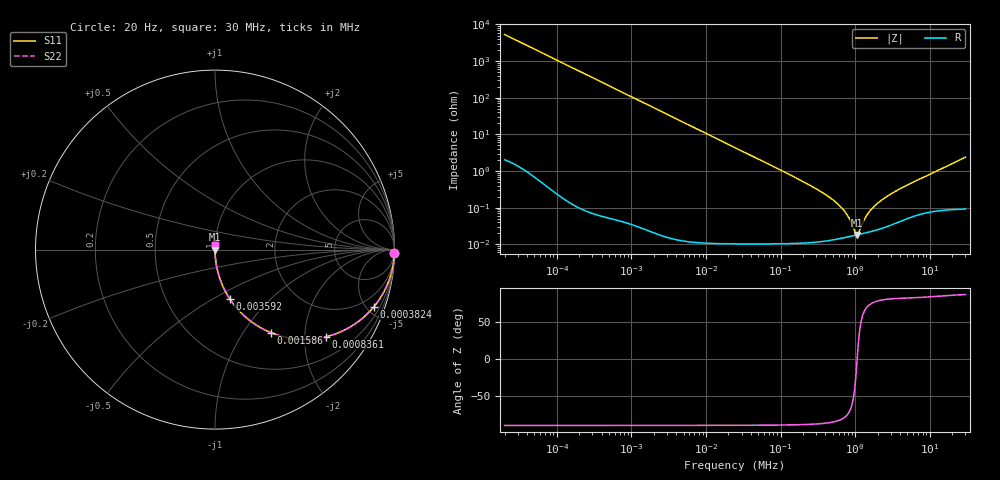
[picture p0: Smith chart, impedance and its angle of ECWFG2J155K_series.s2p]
!  *** S-Parameter ***
!  Copyright (C) Panasonic Industry
!  Plastic Film Capacitor (ECWFG)
!  Parts No. ECWFG2J155K
!  Connection Mode : Series
!  1  o---||---o  2
!  GND o--------o GND
!  Conditions : Temperature = 20   DC Bias = 0 V
! Frequency Range : 20 Hz  -  30 MHz  [ 401 Steps ]
# Hz S RI R 50
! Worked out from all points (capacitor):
!   401 points, 20 Hz to 30 MHz, reference 50 ohm
!   read as one part in series: C = 1.49 uF near 21.47 Hz
!   lowest |Z| = 18.1 mohm at 1.061 MHz (marker M1)
!   series resonance near 1.062 MHz, so ESL is about 15 nH
!   S11 on the Smith chart (normalised r, x): 20 Hz: open; 382.4 Hz: 1.00, -5.58; 836.1 Hz: 1.00, -2.55; 1.586 kHz: 1.00, -1.35; 3.592 kHz: 1.00, -0.59; 30 MHz: 1.00, +0.05
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20  0.9996 -0.0187  0.000358 0.0187  0.000358 0.0187  0.9996 -0.0187
80.02006  0.9944 -0.0745  0.00561 0.0745  0.00561 0.0745  0.9944 -0.0745
216.5336  0.9604 -0.1948  0.0396 0.1948  0.0396 0.1948  0.9604 -0.1948
382.445  0.8862 -0.3175  0.1138 0.3175  0.1138 0.3175  0.8862 -0.3175
836.0918  0.6198 -0.4853  0.3802 0.4853  0.3802 0.4853  0.6198 -0.4853
1585.543  0.3121 -0.4632  0.6879 0.4632  0.6879 0.4632  0.3121 -0.4632
2344.34  0.1719 -0.3771  0.8281 0.3771  0.8281 0.3771  0.1719 -0.3771
3591.727  0.0813 -0.2731  0.9187 0.2731  0.9187 0.2731  0.0813 -0.2731
8430.8  0.0159 -0.1246  0.9841 0.1246  0.9841 0.1246  0.0159 -0.1246
24494.9  0.002 -0.0435  0.998 0.0435  0.998 0.0435  0.002 -0.0435
265198.4  0.000126 -0.00376  0.9999 0.00376  0.9999 0.00376  0.000126 -0.00376
452037.4  0.00013 -0.00191  0.9999 0.00191  0.9999 0.00191  0.00013 -0.00191
645025.1  0.000146 -0.00102  0.9999 0.00102  0.9999 0.00102  0.000146 -0.00102
798395.3  0.000159 -0.000567  0.9998 0.000567  0.9998 0.000567  0.000159 -0.000567
988233  0.000175 -0.00014  0.9998 0.00014  0.9998 0.00014  0.000175 -0.00014
1061060  0.000181 -1.57e-06  0.9998 1.57e-06  0.9998 1.57e-06  0.000181 -1.57e-06
1139253  0.000187 0.000137  0.9998 -0.000137  0.9998 -0.000137  0.000187 0.000137
1410138  0.000207 0.000555  0.9998 -0.000555  0.9998 -0.000555  0.000207 0.000555
1625633  0.000222 0.000845  0.9998 -0.000845  0.9998 -0.000845  0.000222 0.000845
2084991  0.000258 0.00139  0.9997 -0.00139  0.9997 -0.00139  0.000258 0.00139
2871218  0.000325 0.0022  0.9997 -0.0022  0.9997 -0.0022  0.000325 0.0022
3e7  0.00147 0.0236  0.9985 -0.0236  0.9985 -0.0236  0.00147 0.0236
